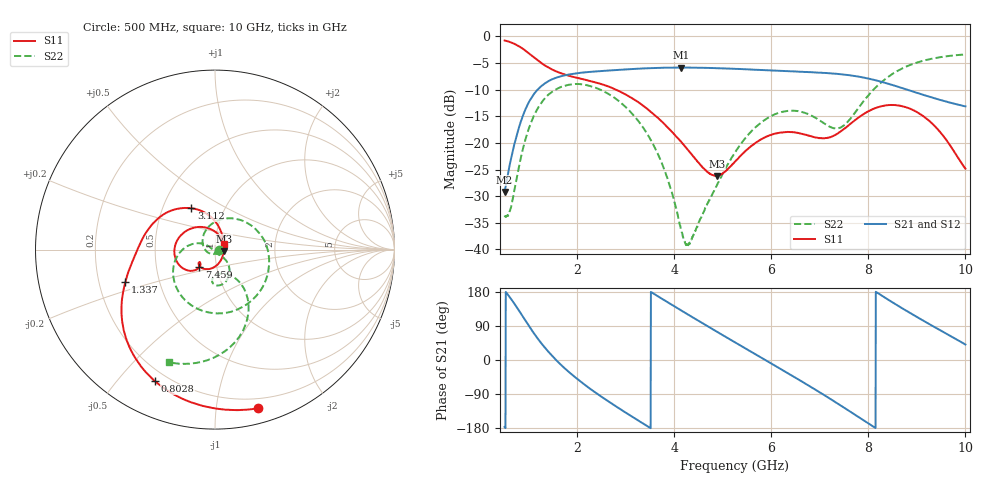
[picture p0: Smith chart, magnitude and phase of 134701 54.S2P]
!  2-Port S-parameters saved by WinCal
! VAR MeasName=S-Parameters (CALIBRATED_DATA) read from VNA (N5242A)
! VAR MeasDate=2013-7-3 16:40:04
! VAR NAME=134701 54
! VAR FILENAME=134701 54.S2P
! VAR DATE=2013-7-3 16:40:04
! VAR PHYS_PORTS=1,2
# Hz S MA R 50
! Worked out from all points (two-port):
!   1601 points, 500 MHz to 10 GHz, reference 50 ohm
!   highest |S21| = -5.84 dB at 4.146 GHz (marker M1); lowest = -29.2 dB at 500 MHz (marker M2)
!   |S21| within 3 dB of the highest: 1.328 GHz to 8.392 GHz (7.064 GHz wide, 145 % of centre)
!   lowest |S11| = -26.2 dB at 4.876 GHz (marker M3), VSWR 1.10, Z = 55.1 - j0.846 ohm
!   |S11| at or under -10 dB: 2.798 GHz to end of sweep
!   |S22| runs from -39.4 to -3.4 dB; largest |S21 - S12| = 0.0024
!   S11 on the Smith chart (normalised r, x): 500 MHz: 0.12, -1.30; 802.8 MHz: 0.15, -0.63; 1.337 GHz: 0.31, -0.16; 3.112 GHz: 0.70, +0.35; 7.459 GHz: 0.82, -0.16; 10 GHz: 1.10, +0.07
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5e8  0.9165 -74.7  0.03456 -176.6  0.03456 -177.1  0.02083 -10.7
6.1875e8  0.8824 -90.9  0.06675 163.4  0.0667 163.2  0.02391 -91.4
8.028125e8  0.8055 -114.6  0.1431 129.1  0.143 128.9  0.0622 170.6
1.105625e9  0.6343 -145.1  0.2882 70.1  0.2879 70.1  0.1806 72.8
1.337188e9  0.5317 -160.0  0.3639 31.5  0.3637 31.4  0.2644 19.7
1.669688e9  0.4498 -175.2  0.4235 -13.7  0.4234 -13.8  0.3364 -37.1
2.085312e9  0.3996 167.7  0.4567 -58.8  0.4557 -59.0  0.3552 -89.3
2.56625e9  0.3483 146.1  0.4757 -102.9  0.4751 -103.0  0.3013 -135.5
3.1125e9  0.2657 119.8  0.4933 -148.2  0.4926 -148.2  0.1921 -176.6
3.670625e9  0.1699 93.3  0.5071 167.4  0.5063 167.4  0.07686 154.5
3.92e9  0.1314 81.6  0.5092 147.9  0.5092 147.9  0.03763 152.4
4.145625e9  0.1017 69.6  0.5104 130.4  0.5097 130.5  0.0148 177.9
4.311875e9  0.08284 58.8  0.5096 117.7  0.5093 117.8  0.01134 -119.7
4.875938e9  0.04904 -9.0  0.5031 74.7  0.5032 74.8  0.03997 -49.0
5.25e9  0.06673 -59.8  0.4963 46.6  0.4966 46.6  0.0815 -44.0
6.004062e9  0.1197 -114.3  0.4793 -9.6  0.4791 -9.7  0.1797 -67.6
6.835312e9  0.1151 -141.3  0.4612 -72.7  0.4612 -72.7  0.1798 -95.1
7.45875e9  0.131 -131.7  0.4402 -122.6  0.441 -122.5  0.1423 -69.9
7.93375e9  0.1904 -142.4  0.4079 -162.0  0.4083 -162.1  0.2576 -53.1
8.420625e9  0.2267 -169.7  0.3582 158.2  0.3577 157.9  0.4216 -64.6
9.228125e9  0.165 131.3  0.2743 96.8  0.2735 96.6  0.6063 -91.5
1e10  0.05734 33.3  0.2206 40.9  0.2194 40.8  0.6774 -112.1
